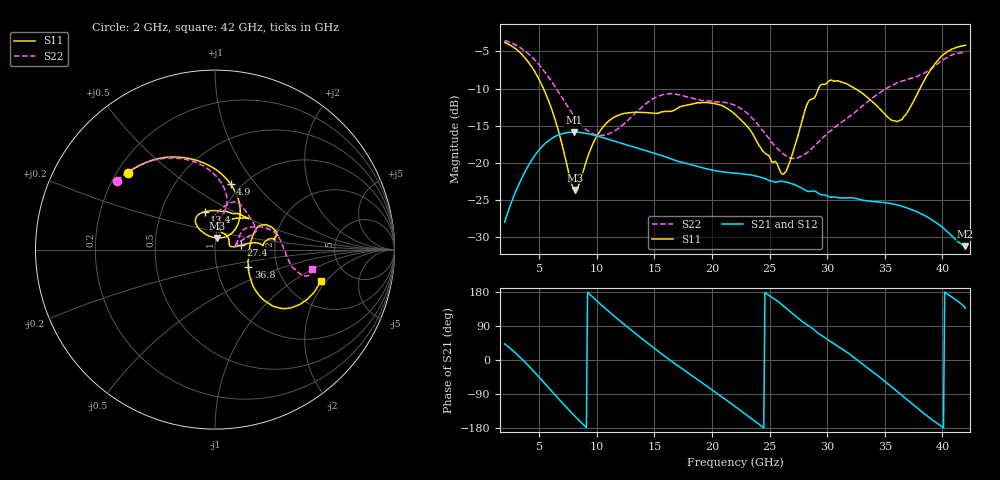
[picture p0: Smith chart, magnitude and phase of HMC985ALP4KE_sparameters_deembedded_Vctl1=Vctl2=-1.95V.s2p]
!s2p File: Measurements: S11, S21, S12, S22
# GHz S dB R 50.0
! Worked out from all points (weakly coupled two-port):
!   401 points, 2 GHz to 42 GHz, reference 50 ohm
!   highest |S21| = -15.86 dB at 8 GHz (marker M1); lowest = -31.2 dB at 42 GHz (marker M2)
!   lowest |S11| = -23.6 dB at 8.1 GHz (marker M3), VSWR 1.14, Z = 50.5 + j6.6 ohm
!   |S11| at or under -10 dB: 5.372 GHz to 29.25 GHz (23.88 GHz wide, 138 % of centre); 32.41 GHz to 38.05 GHz (5.641 GHz wide, 16 % of centre)
!   |S22| runs from -19.4 to -3.5 dB; largest |S21 - S12| = 0.00015
!   S11 on the Smith chart (normalised r, x): 2 GHz: 0.24, +0.36; 4.9 GHz: 0.89, +0.76; 13.4 GHz: 0.82, +0.36; 27.4 GHz: 1.33, +0.06; 36.8 GHz: 1.42, -0.29; 42 GHz: 3.14, -1.79
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2  -3.78 138.4  -27.98 42.7  -27.98 42.8  -3.53 144.9
3.4  -5.26 109.7  -22.34 5.4  -22.34 5.4  -4.56 121.3
4.9  -8.50 76.7  -18.43 -42.1  -18.44 -42.1  -6.63 97.2
6.1  -12.84 52.6  -16.70 -82.9  -16.70 -82.9  -9.11 81.9
8  -23.47 75.2  -15.86 -145.1  -15.87 -145.1  -13.62 76.6
8.1  -23.64 81.6  -15.87 -148.2  -15.87 -148.3  -13.83 77.1
8.7  -21.77 112.9  -15.94 -166.5  -15.94 -166.5  -14.98 81.8
10.6  -15.07 126.5  -16.63 139.7  -16.64 139.7  -16.27 97.5
13.4  -13.19 105.3  -17.95 68.9  -17.95 68.9  -13.22 83.7
15.4  -13.28 79.7  -18.92 21.6  -18.92 21.6  -10.99 69.9
18.9  -11.93 43.9  -20.55 -54.9  -20.55 -54.9  -11.51 44.4
22  -13.45 55.3  -21.38 -122.5  -21.39 -122.5  -12.28 23.0
24.5  -18.53 79.3  -22.06 -179.3  -22.07 -179.3  -15.82 19.3
26.1  -21.50 19.1  -22.48 145.3  -22.48 145.3  -18.68 11.1
27.4  -16.73 9.4  -23.09 112.2  -23.09 112.1  -19.35 8.2
28.7  -11.40 4.9  -23.79 83.9  -23.79 83.9  -18.01 16.8
31.1  -9.05 17.3  -24.71 32.9  -24.71 32.9  -14.69 34.6
33.3  -10.94 28.1  -25.07 -15.7  -25.08 -15.7  -12.08 30.3
35.4  -14.01 8.2  -25.44 -66.2  -25.44 -66.1  -9.79 20.2
36.8  -13.55 -27.7  -26.00 -101.1  -26.00 -101.2  -8.84 10.9
39.7  -6.03 -41.1  -28.29 -170.3  -28.28 -170.4  -6.55 -15.1
42  -4.17 -16.5  -31.20 136.5  -31.22 136.5  -5.21 -11.2
